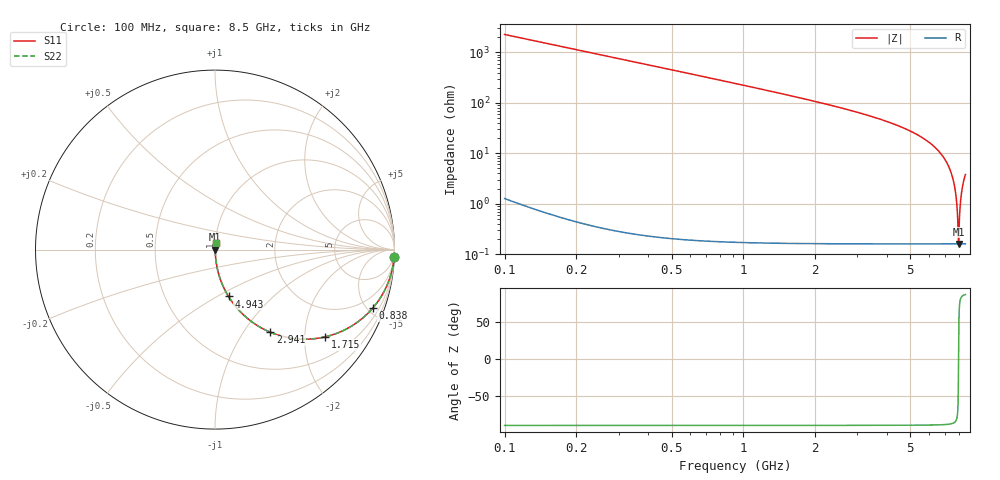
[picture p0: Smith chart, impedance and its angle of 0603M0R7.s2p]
! Created Wed Apr 18 11:59:52 2012
# hz S ma R 50
! 2 Port Network Data from SP1.SP block
! freq  magS11  angS11  magS21  angS21  magS12  angS12  magS22  angS22
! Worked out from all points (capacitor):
!   8401 points, 100 MHz to 8.5 GHz, reference 50 ohm
!   read as one part in series: C = 700 fF near 142 MHz
!   lowest |Z| = 160 mohm at 7.958 GHz (marker M1)
!   series resonance near 7.958 GHz, so ESL is about 570 pH
!   S11 on the Smith chart (normalised r, x): 100 MHz: 1, -45; 838 MHz: 1.00, -5.37; 1.715 GHz: 1.00, -2.53; 2.941 GHz: 1.00, -1.34; 4.943 GHz: 1.00, -0.57; 8.5 GHz: 1.00, +0.08
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1e8  0.999 -2.5  0.04395 87.4  0.04395 87.4  0.999 -2.5
2.24e8  0.9951 -5.6  0.09812 84.3  0.09812 84.3  0.9951 -5.6
3.67e8  0.9871 -9.2  0.1597 80.8  0.1597 80.8  0.9871 -9.2
8.38e8  0.9368 -20.4  0.3492 69.5  0.3492 69.5  0.9368 -20.4
1.5e9  0.825 -34.4  0.5643 55.6  0.5643 55.6  0.825 -34.4
1.715e9  0.7838 -38.3  0.62 51.6  0.62 51.6  0.7838 -38.3
2.9e9  0.5618 -55.7  0.826 34.2  0.826 34.2  0.5618 -55.7
2.941e9  0.5547 -56.2  0.8307 33.7  0.8307 33.7  0.5547 -56.2
4.3e9  0.3503 -69.2  0.9351 20.5  0.9351 20.5  0.3503 -69.2
4.943e9  0.2717 -73.9  0.9609 15.8  0.9609 15.8  0.2717 -73.9
5.7e9  0.1906 -78.5  0.9801 11.0  0.9801 11.0  0.1906 -78.5
7.1e9  0.06523 -84.9  0.9963 3.7  0.9963 3.7  0.06523 -84.9
7.458e9  0.03712 -85.4  0.9977 2.1  0.9977 2.1  0.03712 -85.4
7.699e9  0.01898 -84.1  0.9982 1.1  0.9982 1.1  0.01898 -84.1
7.835e9  0.009037 -79.3  0.9984 0.5  0.9984 0.5  0.009037 -79.3
7.932e9  0.002449 -49.3  0.9984 0.1  0.9984 0.1  0.002449 -49.3
7.958e9  0.001595 0.5  0.9984 -0.0  0.9984 -0.0  0.001595 0.5
7.985e9  0.00252 50.6  0.9984 -0.1  0.9984 -0.1  0.00252 50.6
8.063e9  0.007679 77.6  0.9984 -0.4  0.9984 -0.4  0.007679 77.6
8.149e9  0.01367 82.5  0.9983 -0.8  0.9983 -0.8  0.01367 82.5
8.301e9  0.02421 84.8  0.9981 -1.4  0.9981 -1.4  0.02421 84.8
8.5e9  0.03775 85.4  0.9977 -2.2  0.9977 -2.2  0.03775 85.4
